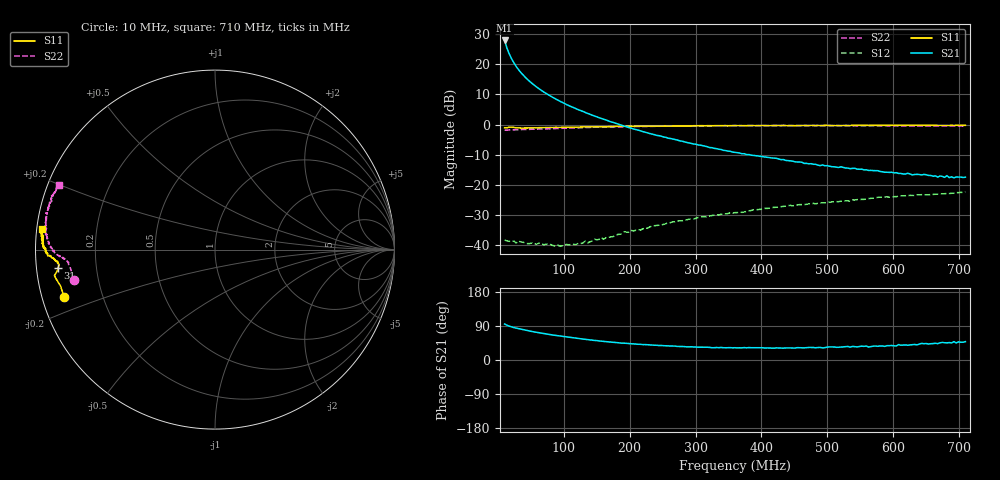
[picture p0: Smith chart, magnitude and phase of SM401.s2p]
!  POLYFET RF DEVICES
!  S PARAMETERS FOR
!  SM401
!  VDS=28, IDQ=800MA
! Date: Wed Jan 23 11:20:25 2002
! SCATTERING PARAMETERS :
# MHZ S MA R 50
! Freq=Mhz Mag[s11] Ang[s11] Mag[s21] Ang[s21] Mag[s12] Ang[s12] Mag[s22] Ang[s22]
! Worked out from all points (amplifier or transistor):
!   201 points, 10 MHz to 710 MHz, reference 50 ohm
!   highest |S21| = 28.0 dB at 10 MHz (marker M1)
!   |S21| within 3 dB of that: start of sweep to 14.37 MHz
!   unconditionally stable (mu >= 1): 84.68 MHz to 209.3 MHz; 210.6 MHz to 222.7 MHz; 500.5 MHz to end of sweep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
!   at 125.5 MHz: K = 1.18, MAG = 19.5 dB, |S12| = -39.6 dB
!   at 360 MHz: K = 0.87, MSG = 10.0 dB, |S12| = -29.3 dB
!   at 710 MHz: K = 1.23, MAG = -0.5 dB, |S12| = -22.4 dB
!   S11 on the Smith chart (normalised r, x): 10 MHz: 0.06, -0.15; 31 MHz: 0.06, -0.06; 710 MHz: 0.02, +0.06
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10  0.8817 -162.4  25.08 95.0  0.01188 9.2  0.8038 -167.7
13.5  0.8838 -166.7  18.77 91.8  0.01157 8.4  0.809 -170.4
17  0.9 -169.5  15.01 89.4  0.01136 7.7  0.8112 -172.3
20.5  0.9064 -170.8  12.51 87.3  0.01135 8.4  0.8142 -173.4
24  0.8923 -171.9  10.69 85.6  0.01146 11.9  0.8182 -174.0
27.5  0.8803 -172.8  9.29 84.2  0.01063 7.2  0.8205 -174.5
31  0.8808 -173.4  8.24 82.7  0.0115 9.0  0.8187 -175.0
34.5  0.8742 -174.0  7.368 81.4  0.01108 11.6  0.8232 -175.2
38  0.8735 -174.6  6.683 80.0  0.01102 10.3  0.8277 -175.5
45  0.8748 -174.8  5.592 77.5  0.01041 11.3  0.8288 -175.8
55.5  0.8821 -175.5  4.469 74.0  0.01033 14.2  0.8367 -176.3
66  0.8883 -175.8  3.687 70.9  0.01047 20.1  0.842 -176.6
76.5  0.8926 -176.1  3.113 67.9  0.01013 22.7  0.8532 -177.0
94  0.8931 -176.4  2.442 63.2  0.00944 32.6  0.8617 -177.5
108  0.9005 -176.8  2.054 59.9  0.00988 40.1  0.8737 -177.9
129  0.9094 -177.2  1.651 55.3  0.01065 51.1  0.8881 -178.5
171  0.9246 -177.8  1.112 47.3  0.01342 67.3  0.9121 179.4
244.5  0.9425 -179.6  0.6518 38.2  0.021 80.0  0.9381 176.3
360  0.9583 178.3  0.3441 32.4  0.03418 85.9  0.9579 170.9
479  0.9657 176.1  0.2179 33.0  0.04871 86.8  0.9618 166.0
594.5  0.9702 174.8  0.1595 37.7  0.06196 86.5  0.9502 161.5
710  0.9692 173.1  0.1329 48.5  0.07582 87.9  0.9418 157.6
